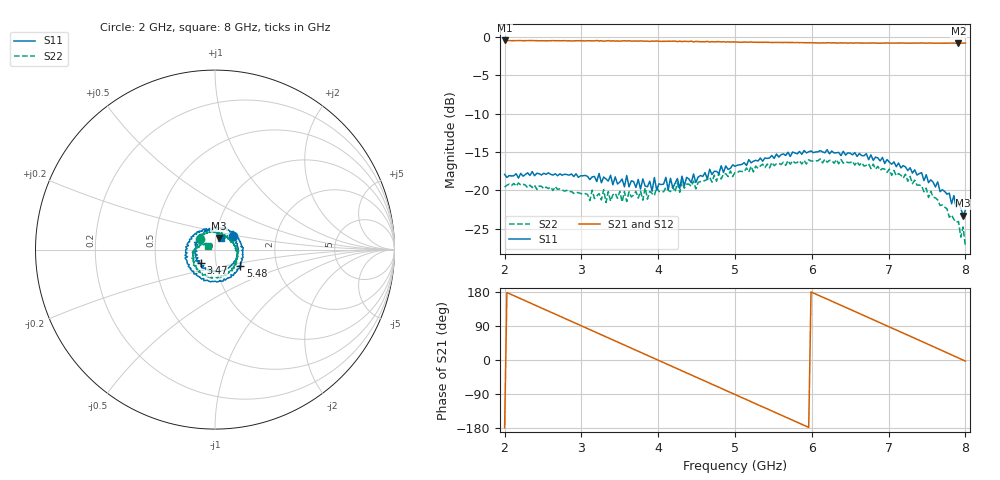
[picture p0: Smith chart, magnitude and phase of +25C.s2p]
!Agilent Technologies,E8361C,US49010292,A.09.42.06
!Agilent E8361C: A.09.42.06
!Date: Tuesday, January 14, 2025 01:18:51
!Correction: S11(Full 2 Port(1,2))
!S21(Full 2 Port(1,2))
!S12(Full 2 Port(1,2))
!S22(Full 2 Port(1,2))
!S2P File: Measurements: S11, S21, S12, S22:
# Hz S  dB  R 50
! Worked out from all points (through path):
!   201 points, 2 GHz to 8 GHz, reference 50 ohm
!   highest |S21| = -0.46 dB at 2 GHz (marker M1); lowest = -0.8 dB at 7.91 GHz (marker M2)
!   group delay of S21, straight-line fit = 251 ps
!   lowest |S11| = -23.3 dB at 7.97 GHz (marker M3), VSWR 1.15, Z = 51.8 + j6.71 ohm
!   |S11| at or under -10 dB: start of sweep to end of sweep
!   |S22| runs from -27.3 to -15.9 dB; largest |S21 - S12| = 0.0077
!   S11 on the Smith chart (normalised r, x): 2 GHz: 1.21, +0.19; 3.47 GHz: 0.84, -0.13; 5.48 GHz: 1.30, -0.25; 8 GHz: 1.06, +0.14
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2e9  -17.93 38.0  -0.46 -179.3  -0.48 -179.2  -19.59 145.3
2.3e9  -17.72 1.9  -0.49 153.5  -0.50 153.6  -19.67 127.8
2.6e9  -17.92 -30.9  -0.50 126.4  -0.49 126.4  -19.57 106.8
3.02e9  -18.12 -78.8  -0.52 88.3  -0.52 88.3  -20.48 84.3
3.47e9  -19.19 -136.5  -0.53 47.6  -0.54 47.4  -21.05 67.1
3.77e9  -19.84 -174.8  -0.52 20.6  -0.58 20.4  -20.13 44.5
4.01e9  -19.16 153.2  -0.56 -1.3  -0.58 -1.4  -20.16 37.1
4.28e9  -19.78 114.0  -0.56 -25.9  -0.60 -25.9  -20.26 25.4
4.31e9  -18.16 112.7  -0.61 -28.7  -0.61 -28.6  -18.87 23.6
4.61e9  -17.70 70.3  -0.63 -55.7  -0.59 -55.7  -18.71 2.5
5e9  -16.87 23.4  -0.67 -91.1  -0.67 -91.0  -17.69 -18.7
5.48e9  -15.47 -33.0  -0.73 -134.4  -0.73 -134.5  -16.37 -50.6
5.75e9  -15.02 -59.2  -0.74 -158.9  -0.77 -158.9  -16.15 -68.2
6.02e9  -15.10 -89.7  -0.78 176.8  -0.77 176.8  -16.19 -88.7
6.29e9  -15.13 -119.2  -0.76 152.5  -0.80 152.5  -16.48 -107.1
6.59e9  -15.58 -149.6  -0.78 125.3  -0.81 125.5  -16.28 -131.0
7.01e9  -16.34 163.8  -0.81 87.3  -0.83 87.5  -17.25 -159.6
7.43e9  -17.69 118.0  -0.81 49.2  -0.82 49.4  -19.40 171.7
7.91e9  -21.56 74.7  -0.83 5.2  -0.81 5.3  -24.07 146.1
7.94e9  -22.33 67.3  -0.80 2.6  -0.82 2.5  -26.11 157.3
7.97e9  -23.33 71.1  -0.82 -0.1  -0.82 -0.2  -24.78 147.9
8e9  -22.58 63.2  -0.80 -2.9  -0.81 -2.9  -27.29 149.3
